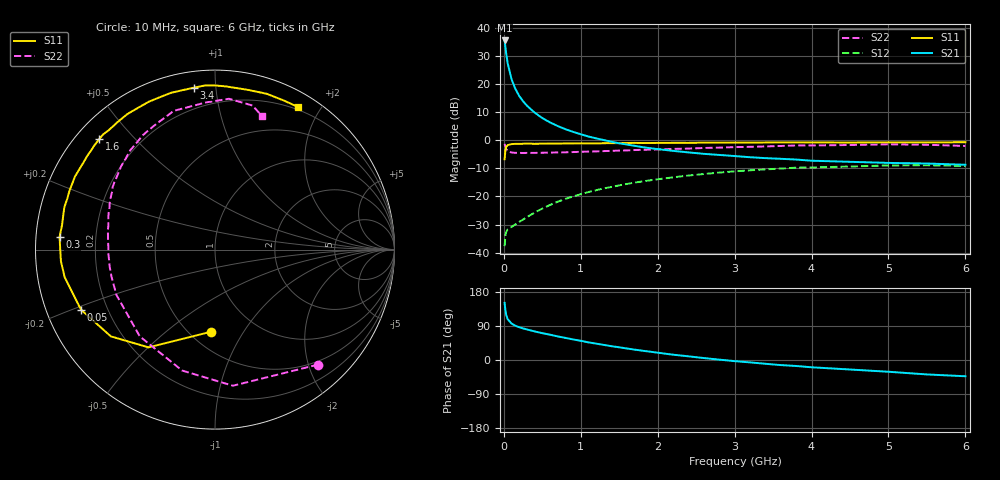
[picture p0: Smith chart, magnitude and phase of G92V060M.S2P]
! SIEMENS Small Signal Semiconductors
! BFG235
! Si NPN RF Bipolar Junction Transistor in SOT223
! VCE = 2 V  IC = 60 mA
! Common Emitter S-Parameters:  July  1994
# GHz  S  MA  R  50
!  f  S11  S21  S12  S22
! GHz  MAG  ANG  MAG  ANG  MAG  ANG  MAG  ANG
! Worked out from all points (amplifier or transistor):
!   40 points, 10 MHz to 6 GHz, reference 50 ohm
!   highest |S21| = 35.4 dB at 10 MHz (marker M1)
!   |S21| within 3 dB of that: start of sweep to 23.23 MHz
!   unconditionally stable (mu >= 1): 469.4 MHz to 1.526 GHz
!   at 200 MHz: K = 0.71, MSG = 22.4 dB, |S12| = -29.0 dB
!   at 1.5 GHz: K = 1.00, MAG = 7.1 dB, |S12| = -16.0 dB
!   at 6 GHz: K = 0.94, MSG = 0.2 dB, |S12| = -9.2 dB
!   S11 on the Smith chart (normalised r, x): 10 MHz: 0.63, -0.73; 50 MHz: 0.10, -0.21; 300 MHz: 0.07, +0.04; 1.6 GHz: 0.07, +0.40; 3.4 GHz: 0.08, +0.88; 6 GHz: 0.17, +1.73
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0.01  0.4584 -92.8  59.11 150.9  0.0131 61.7  0.8605 -48.1
0.02  0.6587 -124.2  45.48 131.6  0.0202 46.1  0.765 -82.5
0.03  0.7553 -140.2  35.14 119.9  0.0233 38.1  0.6983 -105.2
0.05  0.8183 -155.9  23.16 107.8  0.0262 29.9  0.6398 -130.9
0.1  0.8518 -169.7  12.15 96.2  0.0289 29.9  0.6045 -155.3
0.15  0.861 -175.8  8.156 90.5  0.0319 34.9  0.596 -165.2
0.2  0.8614 -179.2  6.102 86.6  0.0353 39.0  0.5947 -170.6
0.25  0.8647 177.8  4.917 83.3  0.0389 43.3  0.5928 -174.3
0.3  0.8687 175.3  4.106 80.6  0.043 46.5  0.5945 -177.3
0.4  0.8631 170.9  3.091 75.4  0.0518 51.0  0.5944 178.6
0.5  0.8667 167.3  2.471 70.8  0.0608 53.3  0.5982 175.3
0.6  0.8719 164.3  2.069 66.8  0.0707 54.8  0.6015 172.4
0.7  0.8706 160.7  1.787 62.2  0.0807 55.4  0.6067 169.7
0.8  0.8745 158.1  1.568 58.3  0.0907 55.2  0.609 167.3
1.1  0.8783 148.9  1.161 46.5  0.1198 52.7  0.6276 160.6
1.6  0.8916 136.4  0.837 30.4  0.1671 45.4  0.6583 150.3
2.2  0.8993 122.9  0.646 14.0  0.2189 34.9  0.6997 138.3
3.2  0.9065 101.6  0.498 -6.3  0.2917 15.7  0.7621 118.7
3.4  0.9097 97.4  0.48 -10.0  0.3024 11.6  0.7746 114.5
4.5  0.9086 78.4  0.413 -25.1  0.3408 -8.9  0.8213 93.6
5.5  0.9147 65.4  0.385 -38.1  0.359 -26.8  0.8294 75.4
6  0.9198 59.8  0.366 -42.9  0.3481 -33.5  0.7894 70.7
